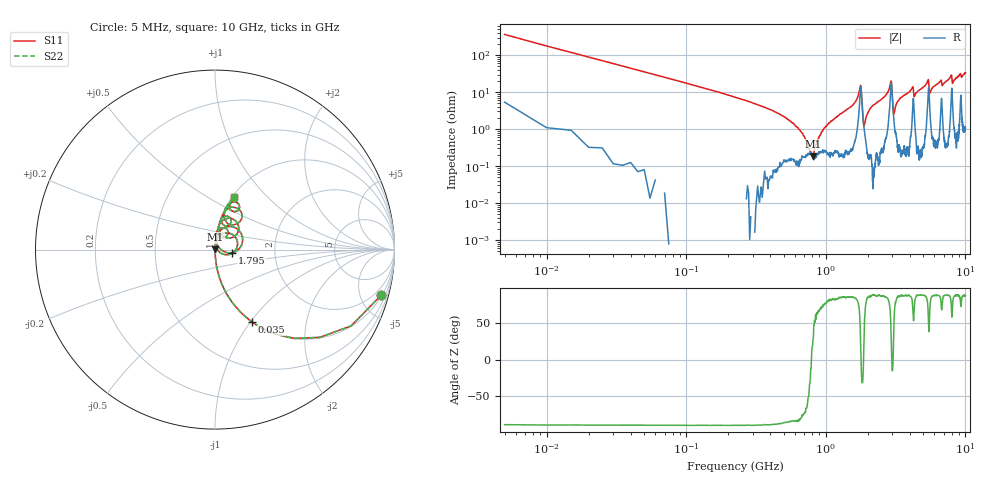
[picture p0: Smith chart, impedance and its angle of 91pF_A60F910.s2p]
! Amotech Co.,Ltd.
! http://www.amotech.co.kr/
! Part Number: A60F910
! These Parameters are Measured in Series Mode Connection
! Operation Temp=25[degC], DC Bias Voltage=0[V]
! Freq. Start=5[MHz] Stop=10[GHz], 2000[Steps]
! Date: Monday, July 20, 2020, 04:40:32
# GHZ S RI R 50.000000
!Freq.(Hz) S11(Real) S11(Imag) S21(Real) S21(Imag) S12(Real) S12(Imag) S22(Real) S22(Imag)
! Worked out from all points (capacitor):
!   2000 points, 5 MHz to 10 GHz, reference 50 ohm
!   read as one part in series: C = 89.2 pF near 55 MHz
!   lowest |Z| = 182 mohm at 805 MHz (marker M1)
!   series resonance near 788.6 MHz, so ESL is about 460 pH
!   S11 on the Smith chart (normalised r, x): 5 MHz: 1.11, -7.27; 35 MHz: 1.00, -1.02; 1.795 GHz: 1.21, -0.05; 10 GHz: 1.02, +0.67
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0.005  0.9264 -0.2538  0.0736 0.2538  0.0736 0.2538  0.9264 -0.2538
0.035  0.2058 -0.4033  0.7942 0.4033  0.7942 0.4033  0.2058 -0.4033
0.12  0.0204 -0.1422  0.9796 0.1422  0.9796 0.1422  0.0204 -0.1422
0.605  0.00139 -0.0125  0.9986 0.0125  0.9986 0.0125  0.00139 -0.0125
0.805  0.0017 0.000646  0.9983 -0.000646  0.9983 -0.000646  0.0017 0.000646
1.03  0.00229 0.0132  0.9977 -0.0132  0.9977 -0.0132  0.00229 0.0132
1.675  0.0133 0.0645  0.9867 -0.0645  0.9867 -0.0645  0.0133 0.0645
1.75  0.0672 0.0938  0.9328 -0.0938  0.9328 -0.0938  0.0672 0.0938
1.795  0.0969 -0.0198  0.9031 0.0198  0.9031 0.0198  0.0969 -0.0198
1.855  0.0164 -0.00428  0.9836 0.00428  0.9836 0.00428  0.0164 -0.00428
1.9  0.00755 0.0118  0.9925 -0.0118  0.9925 -0.0118  0.00755 0.0118
2.115  0.00316 0.0388  0.9968 -0.0388  0.9968 -0.0388  0.00316 0.0388
2.91  0.1043 0.125  0.8957 -0.125  0.8957 -0.125  0.1043 0.125
3.075  0.0177 0.018  0.9823 -0.018  0.9823 -0.018  0.0177 0.018
3.34  0.00755 0.061  0.9925 -0.061  0.9925 -0.061  0.00755 0.061
4.17  0.0408 0.1215  0.9592 -0.1215  0.9592 -0.1215  0.0408 0.1215
5.005  0.0218 0.1344  0.9782 -0.1344  0.9782 -0.1344  0.0218 0.1344
5.395  0.0986 0.1709  0.9014 -0.1709  0.9014 -0.1709  0.0986 0.1709
5.56  0.039 0.0807  0.961 -0.0807  0.961 -0.0807  0.039 0.0807
6.67  0.0691 0.186  0.9309 -0.186  0.9309 -0.186  0.0691 0.186
8.335  0.0524 0.2014  0.9476 -0.2014  0.9476 -0.2014  0.0524 0.2014
10  0.1076 0.2944  0.8924 -0.2944  0.8924 -0.2944  0.1076 0.2944
